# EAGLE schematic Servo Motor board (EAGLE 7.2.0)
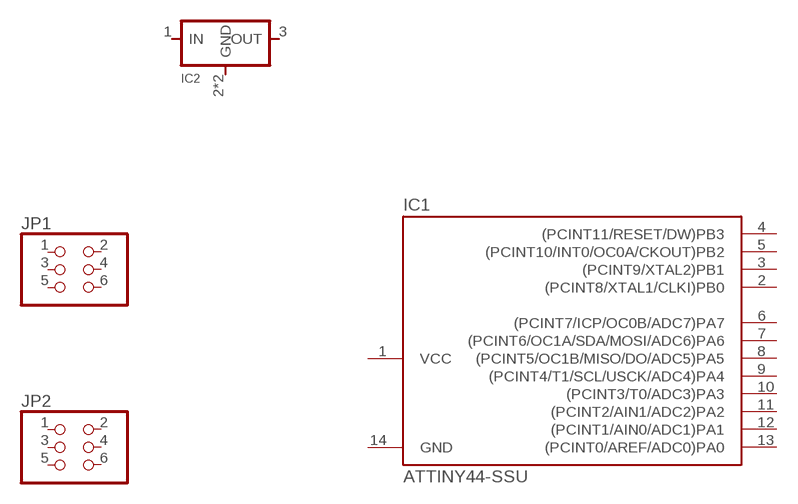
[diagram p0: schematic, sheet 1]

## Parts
IC1  ATTINY44-SSU  [SOIC14]
IC2  REGULATORSOT223  [SOT223]
JP1  PINHD-2X3-SMD  [2X03SMD]
JP2  PINHD-2X3-SMD  [2X03SMD]
Unconnected: IC1.2((PCINT8/XTAL1/CLKI)PB0) IC1.3((PCINT9/XTAL2)PB1) IC1.4((PCINT11/RESET/DW)PB3) IC1.5((PCINT10/INT0/OC0A/CKOUT)PB2) IC1.6((PCINT7/ICP/OC0B/ADC7)PA7) IC1.7((PCINT6/OC1A/SDA/MOSI/ADC6)PA6) IC1.8((PCINT5/OC1B/MISO/DO/ADC5)PA5) IC1.9((PCINT4/T1/SCL/USCK/ADC4)PA4) IC1.10((PCINT3/T0/ADC3)PA3) IC1.11((PCINT2/AIN1/ADC2)PA2) IC1.12((PCINT1/AIN0/ADC1)PA1) IC1.13((PCINT0/AREF/ADC0)PA0) IC2.1(IN) IC2.2(GND) IC2.3(OUT) IC2.4(GND) JP1.1 JP1.2 JP1.3 JP1.4 JP1.5 JP1.6 JP2.1 JP2.2 JP2.3 JP2.4 JP2.5 JP2.6

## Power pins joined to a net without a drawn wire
GND: IC1.14(GND)
VCC: IC1.1(VCC)

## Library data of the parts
IC1 = 01_fab:ATTINY44
IC2 = 01_fab:REGULATOR
JP1 JP2 = 01_fab:PINHD-2X3-SMD: PIN HEADER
